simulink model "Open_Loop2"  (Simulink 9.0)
settings: Solver=ode45  StartTime=0.0  StopTime=300  RelTol=1e-3  EnableMultiTasking=on
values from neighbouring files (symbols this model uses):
  Cza = -0.032    [init.m]    (also in init_pitch.m)
  Czde = -0.0087    [init.m]    (also in init_pitch.m)
  d2r = 1/r2d    (= 0.0174532925199)    [freq.m]    (also in init.m; frequ.m; init_lat.m; pl.m)
  Mv = 1219.1    [init.m]    (also in init_lat.m; init_pitch.m)
  Qbar = 1220.6    [init.m]    (also in init_lat.m; init_pitch.m)
  r2d = 180/pi    (= 57.2957795131)    [freq.m]    (also in init.m; frequ.m; init_lat.m; pl.m)
  Sref = 145.4    [init.m]    (also in init_lat.m; init_pitch.m)
undefined symbols (not defined in the file or in its folder): Ap, Bp, Cp, Dp

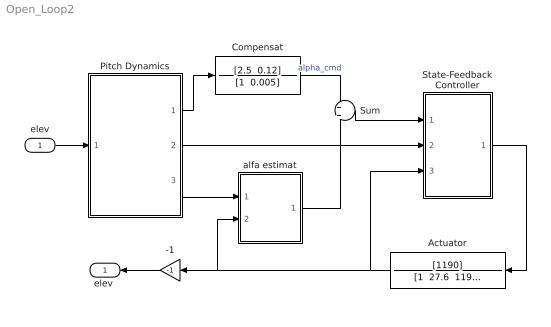
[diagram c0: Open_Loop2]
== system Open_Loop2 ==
  elev : Inport
  -1 : Gain  Gain=-1
  Actuator : TransferFcn  Numerator=[1190]  Denominator="[1  27.6  1190]"
  Compensat : TransferFcn  Numerator="[2.5  0.12]"  Denominator="[1  0.005]"
  Pitch Dynamics : Subsystem
  State-Feedback Controller : Subsystem
  Sum : Sum  Inputs=+|+
  alfa estimat : Subsystem
  "elev " : Outport
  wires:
  Pitch Dynamics/2(q) -> State-Feedback Controller/2(q)
  Sum/1 -> State-Feedback Controller/1(alfa)
  Compensat/1 -> Sum/1  "alpha_cmd"
  State-Feedback Controller/1(delv_cmd) -> Actuator/1
  Actuator/1 -> alfa estimat/2(d-elev), -1/1, State-Feedback Controller/3(d-elev)
  Pitch Dynamics/3(Nz) -> alfa estimat/1(Nz)
  alfa estimat/1(alf_est) -> Sum/2
  elev/1 -> Pitch Dynamics/1(elev)
  Pitch Dynamics/1(gamma) -> Compensat/1
  -1/1 -> "elev "/1

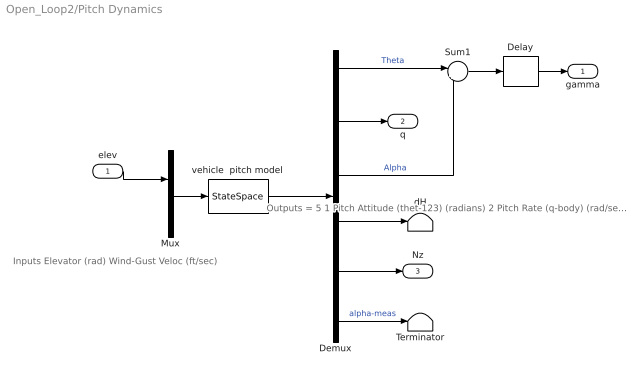
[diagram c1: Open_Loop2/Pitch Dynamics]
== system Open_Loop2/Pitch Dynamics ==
  note: Inputs Elevator (rad) Wind-Gust Veloc (ft/sec)
  note: Outputs = 5 1 Pitch Attitude (thet-123) (radians) 2 Pitch Rate (q-body) (rad/sec) 3 Angle of attack, alfa, (radians) 4 Change in Altitude, delta-H, (feet) 5 Z-Acceleromet, (ft/sec^2) Translation 6 Alpha Sensed at Vane (radian)
  elev : Inport
  Delay : TransportDelay  DelayTime=0.7  PadeOrder=2
  Demux : Demux  Outputs=6
  Mux : Mux  Inputs=2
  Sum1 : Sum  Inputs=|+-
  Terminator : Terminator
  dH : Terminator
  vehicle  pitch model : StateSpace  A=Ap  B=Bp  C=Cp  D=Dp  InitialCondition=0
  gamma : Outport
  q : Outport  Port=2
  Nz : Outport  Port=3
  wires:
  Mux/1 -> vehicle  pitch model/1
  Demux/2 -> q/1
  elev/1 -> Mux/1
  Demux/3 -> Sum1/2  "Alpha"
  Demux/6 -> Terminator/1  "alpha-meas"
  Sum1/1 -> Delay/1
  Demux/1 -> Sum1/1  "Theta"
  Demux/5 -> Nz/1
  Demux/4 -> dH/1
  vehicle  pitch model/1 -> Demux/1
  Delay/1 -> gamma/1

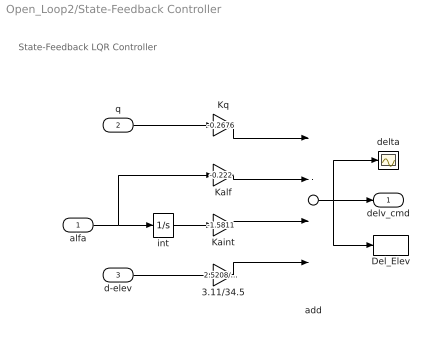
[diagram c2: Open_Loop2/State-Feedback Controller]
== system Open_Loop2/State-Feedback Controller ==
  note: State-Feedback LQR Controller
  alfa : Inport
  q : Inport  Port=2
  d-elev : Inport  Port=3
  3.11/34.5 : Gain  Gain=2.5208/34.5
  Del_Elev : ToWorkspace  VariableName=delev  SampleTime=-1
  Kaint : Gain  Gain=-1.5811
  Kalf : Gain  Gain=-0.222
  Kq : Gain  Gain=-0.2676
  add : Sum  Inputs=----
  delta : Scope
  int : Integrator
  delv_cmd : Outport
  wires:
  alfa/1 -> int/1, Kalf/1
  int/1 -> Kaint/1
  Kq/1 -> add/1
  Kalf/1 -> add/2
  Kaint/1 -> add/3
  3.11/34.5/1 -> add/4
  d-elev/1 -> 3.11/34.5/1
  q/1 -> Kq/1
  add/1 -> delv_cmd/1, delta/1, Del_Elev/1

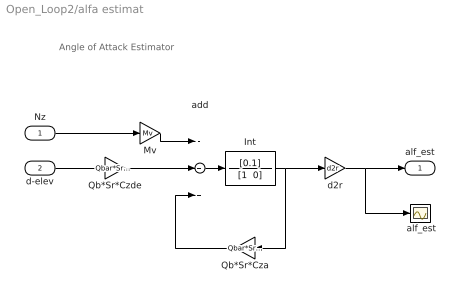
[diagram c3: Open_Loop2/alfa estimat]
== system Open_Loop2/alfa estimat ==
  note: Angle of Attack Estimator
  Nz : Inport
  d-elev : Inport  Port=2
  " alf_est" : Scope
  Int : TransferFcn  Numerator=[0.1]  Denominator="[1  0]"
  Mv : Gain  Gain=Mv
  Qb*Sr*Cza : Gain  Gain=Qbar*Sref*Cza
  Qb*Sr*Czde : Gain  Gain=Qbar*Sref*Czde*r2d
  add : Sum  Inputs=-++
  d2r : Gain  Gain=d2r
  alf_est : Outport
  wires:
  add/1 -> Int/1
  Qb*Sr*Cza/1 -> add/3
  Mv/1 -> add/1
  Qb*Sr*Czde/1 -> add/2
  d2r/1 -> " alf_est"/1, alf_est/1
  Int/1 -> Qb*Sr*Cza/1, d2r/1
  d-elev/1 -> Qb*Sr*Czde/1
  Nz/1 -> Mv/1
